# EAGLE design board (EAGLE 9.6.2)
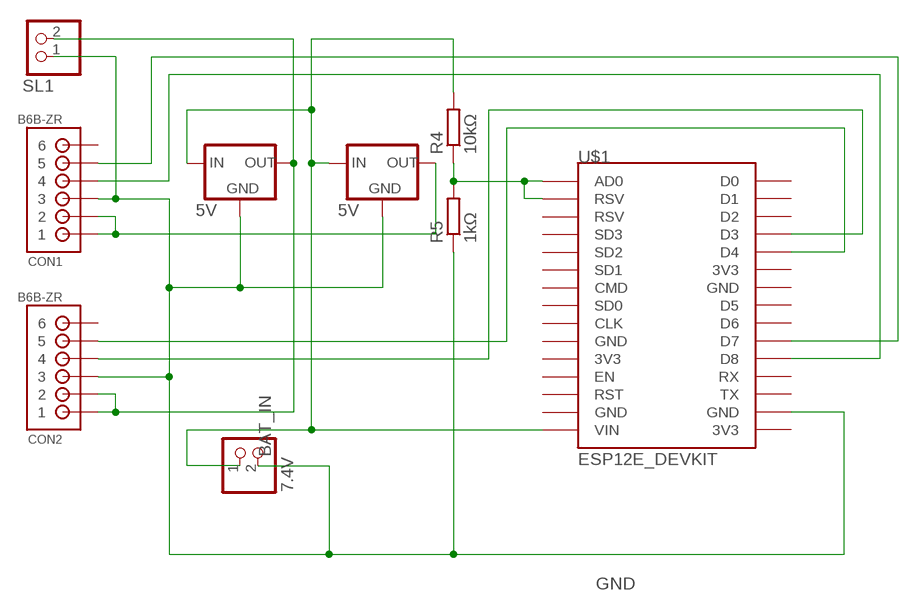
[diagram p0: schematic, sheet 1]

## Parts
BAT_IN  7.4V  PINHD-1X2  [1X02]
CON1  B6B-ZR  [B6B-ZR]
CON2  B6B-ZR  [B6B-ZR]
L78S05CV_1VREGULATOR  5V  78XXS  [78XXS]
L78S05CV_2VREGULATOR  5V  78XXS  [78XXS]
R4  10kΩ  R-EU_0204/7  [0204/7]
R5  1kΩ  R-EU_0204/7  [0204/7]
SL1  PINHD-1X2  [1X02]
U$1  ESP12E_DEVKIT  [ESP12E_DEVKIT]

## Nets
GND: BAT_IN.2 CON1.3 CON2.3 L78S05CV_1VREGULATOR.GND L78S05CV_2VREGULATOR.GND R5.1 SL1.1 U$1.GND@3(GND)
N$1: CON2.1 CON2.2 L78S05CV_2VREGULATOR.OUT SL1.2
N$2: R4.1 R5.2 U$1.AD0 U$1.RSV@0(RSV)
N$3: CON1.1 CON1.2 L78S05CV_1VREGULATOR.OUT
N$4: CON1.5 U$1.D7
N$7: CON2.5 U$1.D4
N$8: CON2.4 U$1.D3
N$10: CON1.4 U$1.D8
VCC: BAT_IN.1 L78S05CV_1VREGULATOR.IN L78S05CV_2VREGULATOR.IN R4.2 U$1.VIN
Unconnected: CON1.6 CON2.6 U$1.3V3@0(3V3) U$1.3V3@1(3V3) U$1.3V3@2(3V3) U$1.CLK U$1.CMD U$1.D0 U$1.D1 U$1.D2 U$1.D5 U$1.D6 U$1.EN U$1.GND@0(GND) U$1.GND@1(GND) U$1.GND@2(GND) U$1.RST U$1.RSV@1(RSV) U$1.RX U$1.SD0 U$1.SD1 U$1.SD2 U$1.SD3 U$1.TX

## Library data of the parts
BAT_IN SL1 = pinhead:PINHD-1X2: PIN HEADER
CON1 CON2 = jst:B6B-ZR: JST-ZH Connector 6 pol, 1.5mm pitch Package: B6B-ZR Source: http://www.jst-mfg.com/product/pdf/eng/eZH.pdf
L78S05CV_1VREGULATOR L78S05CV_2VREGULATOR = v-reg:78XXS: VOLTAGE REGULATOR
R4 R5 = rcl:R-EU_: RESISTOR, European symbol; SPICEPREFIX: R
U$1 = ESP12E_DEVKIT:ESP12E_DEVKIT: ESP12E DEVKIT BOARD

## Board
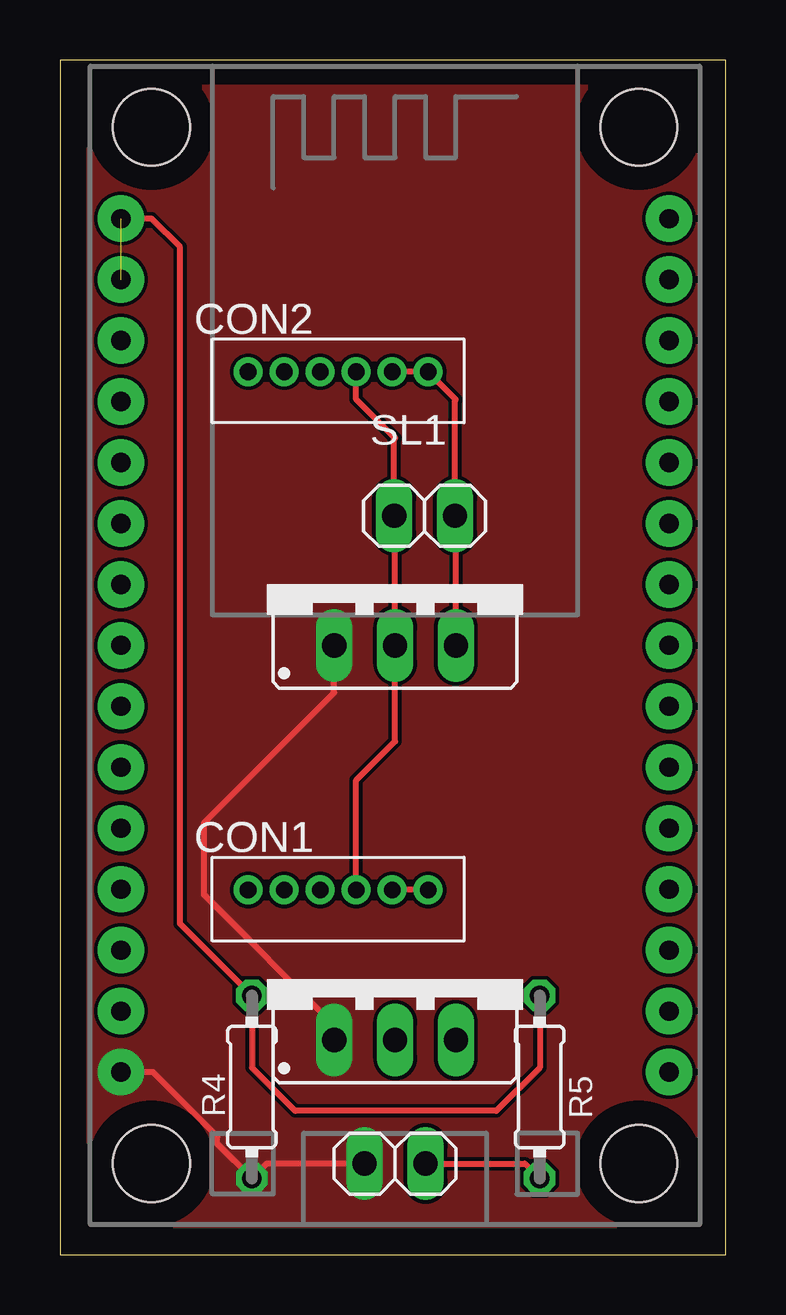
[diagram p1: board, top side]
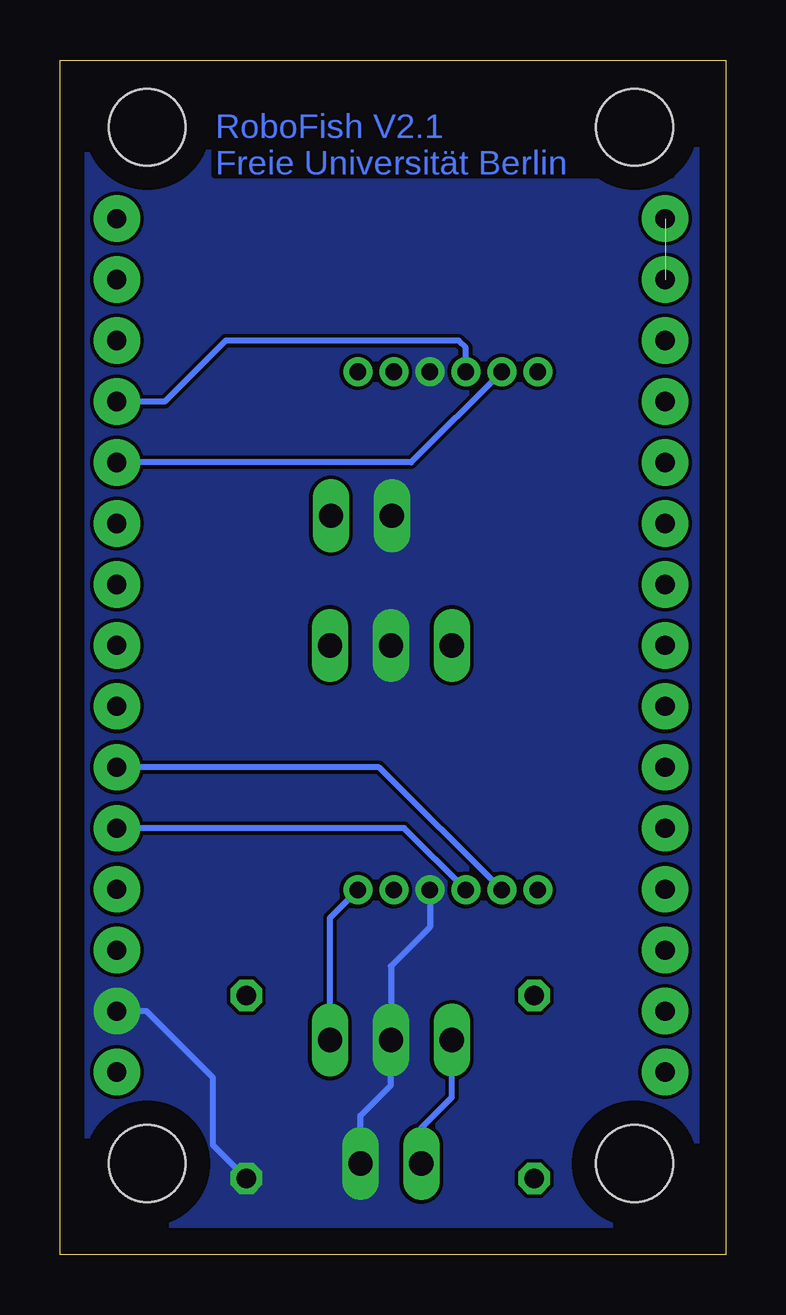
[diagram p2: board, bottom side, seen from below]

Size 27.77 x 49.79 mm. Coordinates in mm from the lower left corner, seen from the top.
Outline: 0,0 27.77,0 27.77,49.79 0,49.79 0,0
Copper layers (1*16): Top 0.035mm / dielectric 1.5mm / Bottom 0.035mm
Design rules "default *": minimum track width 6mil, minimum drill 0.35mm, track to track 6mil, track to pad 6mil, pad to pad 6mil, via to via 6mil, smd to smd 6mil, copper to edge 40mil, drill to drill 6mil, minimum pad ring 10mil, minimum via ring 8mil, stop-mask expansion 4mil, vias tented up to drill 0mil, thermal gap 10mil

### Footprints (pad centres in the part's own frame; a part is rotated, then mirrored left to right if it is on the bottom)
1X02 = drill 1.016 long: 1 -1.27,0; 2 1.27,0
B6B-ZR = drill 0.7: 1 9,-1.3; 2 7.5,-1.3; 3 6,-1.3; 4 4.5,-1.3; 5 3,-1.3; 6 1.5,-1.3
78XXS = drill 1.016 long: GND 0,-2.54; IN -2.54,-2.54; OUT 2.54,-2.54
0204/7 = drill 0.813 octagon: 1 -3.81,0; 2 3.81,0
ESP12E_DEVKIT = drill 0.8 pad 1.93: 3V3@0 -11.43,-7.62; 3V3@1 11.43,5.08; 3V3@2 11.43,-17.78; AD0 -11.43,17.78; CLK -11.43,-2.54; CMD -11.43,2.54; D0 11.43,17.78; D1 11.43,15.24; D2 11.43,12.7; D3 11.43,10.16; D4 11.43,7.62; D5 11.43,0; D6 11.43,-2.54; D7 11.43,-5.08; D8 11.43,-7.62; EN -11.43,-10.16; GND@0 -11.43,-5.08; GND@1 -11.43,-15.24; GND@2 11.43,2.54; GND@3 11.43,-15.24; RST -11.43,-12.7; RSV@0 -11.43,15.24; RSV@1 -11.43,12.7; RX 11.43,-10.16; SD0 -11.43,0; SD1 -11.43,5.08; SD2 -11.43,7.62; SD3 -11.43,10.16; TX 11.43,-12.7; VIN -11.43,-17.78 | hole 3.2: -10.16,21.59; 10.16,21.59; 10.16,-21.59; -10.16,-21.59

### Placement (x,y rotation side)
BAT_IN  13.97,3.81 0 top
CON1  6.35,16.51 0 top
CON2  6.35,38.1 0 top
L78S05CV_1VREGULATOR  13.97,11.49 0 top
L78S05CV_2VREGULATOR  13.97,27.94 0 top
R4  8,7 270 top
R5  20,7 90 top
SL1  15.2,30.8 0 top
U$1  13.97,25.4 0 top

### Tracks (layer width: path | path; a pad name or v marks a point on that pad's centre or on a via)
GND
  Top 0.254: CON2.3 12.35,35.65 13.97,34.03 13.93,33.99 SL1.1 13.97,30.76 L78S05CV_2VREGULATOR.GND 13.97,21.4 12.35,19.78 CON1.3 | BAT_IN.2 19.38,3.81 R5.1
  Bottom 0.254: CON1.3 12.35,13.65 13.97,12.03 L78S05CV_1VREGULATOR.GND 13.97,7.08 15.24,5.81 BAT_IN.2 | R5.1 21.39,4.58 21.39,7.39 24.16,10.16 U$1.GND@3
  pour Bottom (no thermals): 1.27,49.53 26.67,49.53 26.67,1.27 1.27,1.27
N$1
  Top 0.254: CON2.2 CON2.1 16.51,35.64 16.47,35.6 SL1.2 16.51,30.76 L78S05CV_2VREGULATOR.OUT
N$2  (1 unrouted)
  Top 0.254: R5.2 20,7.81 18.19,6 9.81,6 8,7.81 R4.1 5,13.81 5,42 3.82,43.18 U$1.AD0
N$3
  Top 0.254: CON1.1 CON1.2
  Bottom 0.254: L78S05CV_1VREGULATOR.OUT 16.51,14.05 CON1.1
N$4
  Bottom 0.254: CON1.5 14.46,20.32 U$1.D7
N$7
  Bottom 0.254: CON2.5 13.13,33.02 U$1.D4
N$8
  Bottom 0.254: CON2.4 10.85,37.8 11.15,38.1 20.86,38.1 23.4,35.56 U$1.D3
N$10
  Bottom 0.254: CON1.4 13.42,17.78 U$1.D8
VCC
  Top 0.254: BAT_IN.1 8.62,3.81 R4.2 6.55,4.64 6.55,4.95 3.88,7.62 U$1.VIN | L78S05CV_1VREGULATOR.IN 11.43,9.57 6,15 6,18 11.43,23.43 L78S05CV_2VREGULATOR.IN
  Bottom 0.254: BAT_IN.1 12.7,5.3 11.43,6.57 L78S05CV_1VREGULATOR.IN
  pour Top (no thermals): 1.27,49.53 26.67,49.53 26.67,1.27 1.27,1.27

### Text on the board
Bottom: RoboFish V2.1 / Freie Universität Berlin
_tNames: CON2 | CON1 | R4 | R5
